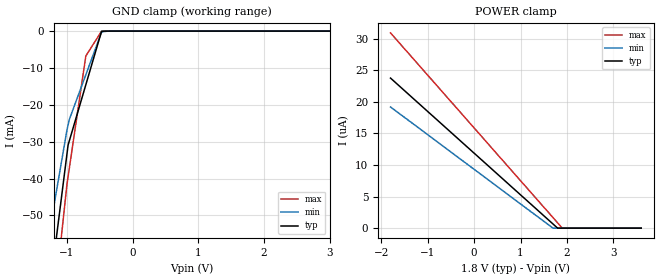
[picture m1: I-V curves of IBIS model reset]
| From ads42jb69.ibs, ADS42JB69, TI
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|   reset Model
[Model]   reset
Model_type   Input
Vinl = 0.4
Vinh = 1.2
|   typ   min   max
|   (nom PVT)   (fast PVT)   (slow PVT)
C_comp   1.280e-12   1.241e-12   1.322e-12
| Where nom  PVT is Nominal Process, 1.8V, 25C
|   Fast PVT is Strong Process,  1.9V, -40C
|   Slow PVT is Weak Process,   1.7V, 125C
[Voltage Range]   1.8   1.7   1.9
|Junction Temperature
[Temperature Range]   25   125   -40
[Power Clamp Reference]   1.8   1.7   1.9
[GND Clamp Reference]   0   0   0
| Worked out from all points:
|   GND clamp passes 1 mA (typ) near -0.49 V on its own axis
[GND Clamp]
|   Voltage   I(typ)   I(min)   I(max)
-1.8V     -820.8mA   -109.7mA   -1.727A
-1.49V    -102.3mA   -77.53mA   -123.3mA
-1.001V   -33.54mA   -26.99mA   -41.79mA
-982.8mV  -30.93mA   -25.47mA   -39.5mA
-965.6mV  -29.89mA   -24.06mA   -37.41mA
-712.5mV  -14.56mA   -11.85mA   -6.75mA
-473.1mV  -74.83uA   -298.8uA   -30.5uA
-280.5mV  -2.29uA    -5.033uA   -2.374uA
3.6V      0A         0A         0A
[POWER Clamp]
|   Voltage   I(typ)   I(min)   I(max)
-1.8V     23.78uA    19.2uA     30.94uA
1.698V    671.7nA    0A         1.687uA
1.798V    11.89nA    0A         851.2nA
1.898V    0A         0A         15.89nA
3.6V      0A         0A         0A
